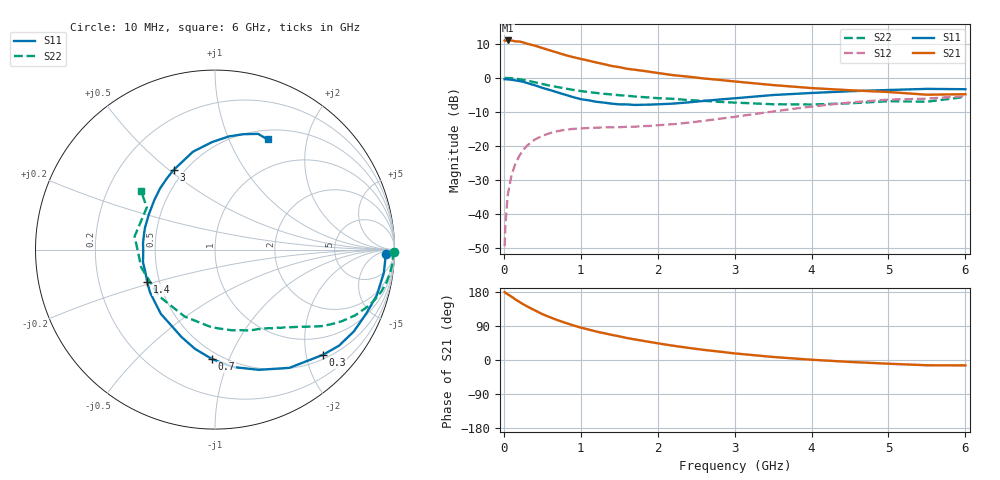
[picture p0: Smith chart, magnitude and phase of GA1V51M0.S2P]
! Infineon Technologies  Discrete & RF Semiconductors
! BF775
! Si NPN RF Bipolar Junction Transistor in SOT23
! VCE = 1.5 V  IC = 1 mA
! Common Emitter S-Parameters:  May  1996
# GHz  S  MA  R  50
!  f  S11  S21  S12  S22
! GHz  MAG  ANG  MAG  ANG  MAG  ANG  MAG  ANG
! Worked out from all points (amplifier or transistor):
!   36 points, 10 MHz to 6 GHz, reference 50 ohm
!   highest |S21| = 11.0 dB at 50 MHz (marker M1)
!   |S21| within 3 dB of that: start of sweep to 613.7 MHz
!   unconditionally stable (mu >= 1): 1.376 GHz to end of sweep
!   at 250 MHz: K = 0.21, MSG = 15.8 dB, |S12| = -21.2 dB
!   at 1.4 GHz: K = 1.02, MAG = 8.2 dB, |S12| = -14.5 dB
!   at 6 GHz: K = 1.06, MAG = -1.3 dB, |S12| = -5.3 dB
!   S11 on the Smith chart (normalised r, x): 10 MHz: 32, -17; 300 MHz: 0.59, -2.34; 700 MHz: 0.45, -0.87; 1.4 GHz: 0.43, -0.19; 3 GHz: 0.44, +0.52; 6 GHz: 0.61, +1.40
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0.01  0.9525 -1.5  3.526 179.1  0.0034 87.4  0.9994 -0.7
0.02  0.9503 -3.2  3.473 177.2  0.007 89.7  0.9888 -1.4
0.05  0.9496 -7.8  3.528 173.5  0.0189 85.5  0.994 -3.7
0.1  0.9367 -15.7  3.527 167.1  0.0376 80.6  0.9846 -7.3
0.15  0.9151 -22.9  3.418 159.9  0.0548 75.1  0.9728 -10.8
0.2  0.8981 -30.5  3.404 153.6  0.0715 71.1  0.956 -14.1
0.25  0.8738 -37.8  3.312 147.4  0.0866 66.4  0.9333 -17.4
0.3  0.8404 -44.2  3.161 141.7  0.101 62.8  0.9117 -20.1
0.4  0.7784 -57.8  2.971 131.4  0.1239 55.5  0.8631 -25.1
0.5  0.7133 -69.9  2.734 121.1  0.1413 49.4  0.811 -29.5
0.7  0.6098 -91.6  2.332 105.1  0.1653 40.3  0.7306 -35.7
0.9  0.5214 -111.0  2.013 91.5  0.1782 34.4  0.6657 -40.2
1.1  0.4682 -130.1  1.786 80.4  0.1837 30.7  0.6177 -44.3
1.4  0.4181 -154.6  1.491 66.4  0.1881 27.8  0.5705 -49.9
1.8  0.4028 174.8  1.269 51.0  0.1955 29.4  0.5225 -57.1
2.2  0.4181 151.6  1.094 37.7  0.2088 32.0  0.4914 -66.6
3  0.5007 117.2  0.884 17.4  0.2679 35.8  0.4332 -92.5
3.5  0.5591 102.7  0.782 8.0  0.3209 33.8  0.4095 -114.5
4.5  0.6354 83.0  0.657 -5.1  0.4346 22.9  0.4227 -166.3
5  0.6625 76.1  0.619 -9.8  0.4787 15.4  0.4539 170.6
5.5  0.688 69.6  0.565 -13.9  0.4944 7.1  0.4465 148.3
6  0.6802 64.5  0.575 -14.2  0.5403 2.7  0.5253 141.6
